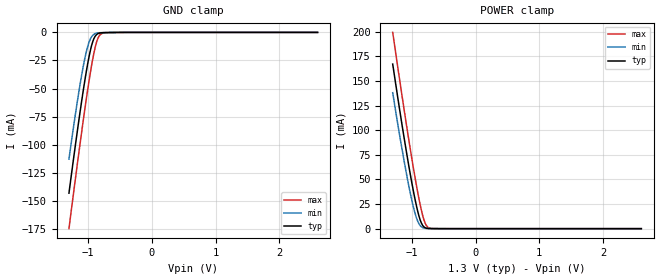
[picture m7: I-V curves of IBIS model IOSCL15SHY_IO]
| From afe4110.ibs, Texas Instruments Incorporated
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|   IOSCL15SHY_IO model
[Model]   IOSCL15SHY_IO
Model_type   Input
Vinl =  0.39V |0.275V for 1.1V
Vinh =  0.91V |0.825V for 1.1V
|   typ   min   max
|   (nom)   (fast)   (weak)
C_comp   0.5884pF   0.4739pF   0.7328pF
[Model Spec]
Vinl   0.39V   0.275V   0.465V
Vinh   0.91V   0.825V   1.085V
[Voltage Range]   1.300V   1.100V   1.550V
[Temperature Range]   27.0   85.0   0.0
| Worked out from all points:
|   GND clamp passes 1 mA (typ) near -0.84 V on its own axis
|   POWER clamp passes 1 mA (typ) near -0.79 V on its own axis
[GND Clamp]
|   Voltage   I(typ)   I(min)   I(max)
-1.3V     -143.2mA   -112.9mA   -174.9mA
-1.222V   -109.9mA   -81.65mA   -140.3mA
-1.143V   -77.79mA   -52.44mA   -106.6mA
-1.084V   -55.04mA   -32.86mA   -82.06mA
-1.026V   -34.2mA    -16.76mA   -58.59mA
-986.4mV  -22.06mA   -8.997mA   -43.83mA
-927.6mV  -8.373mA   -2.67mA    -23.95mA
-868.8mV  -2.028mA   -722.6uA   -9.045mA
-810.1mV  -490.6uA   -271.4uA   -2.024mA
-751.3mV  -214.1uA   -158.1uA   -457.6uA
-535.7mV  -51.28uA   -42.72uA   -66.06uA
2.6V      0A         0A         0A
[POWER Clamp]
|   Voltage   I(typ)   I(min)   I(max)
-1.3V     167mA      138mA      199.2mA
-1.202V   125.3mA    99.03mA    155.8mA
-1.104V   85.44mA    62.67mA    113.6mA
-1.026V   55.67mA    36.46mA    81.32mA
-966.8mV  35.26mA    19.74mA    58.34mA
-908mV    17.72mA    7.569mA    37.01mA
-849.2mV  5.553mA    1.802mA    18.48mA
-810.1mV  1.767mA    597.8uA    8.95mA
-790.5mV  928uA      350.6uA    5.498mA
-751.3mV  267.3uA    139.6uA    1.583mA
-614.1mV  36.92uA    32.58uA    49.79uA
2.6V      0A         0A         0A
